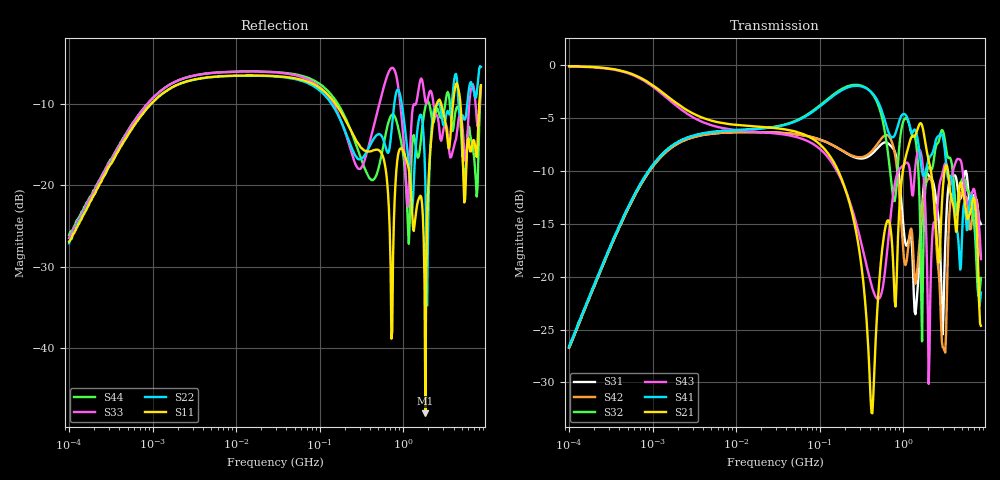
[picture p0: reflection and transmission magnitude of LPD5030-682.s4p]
# MHz S MA R 50
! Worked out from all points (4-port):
!   498 points, 100 kHz to 8.5 GHz, reference 50 ohm
!   strongest paths, dB at 100 kHz, 1.698 MHz, 29.49 MHz, 500.7 MHz, 8.5 GHz:
!     S21: -0.1, -3.3, -5.9, -21.9, -24.6
!     S41: -26.6, -7.6, -5.8, -3.5, -21.5
!     S43: -0.1, -3.5, -6.4, -22.1, -18.3
!     S32: -26.6, -7.6, -5.8, -3.7, -20.1
!     S42: -26.7, -7.8, -6.4, -7.4, -18.2
!     S31: -26.7, -7.8, -6.4, -7.8, -15.0
!   lowest |S11| = -48.1 dB at 1.84 GHz (marker M1), VSWR 1.01, Z = 50.2 - j0.32 ohm
!   |S11| at or under -10 dB: 156.2 MHz to 2.512 GHz (2.356 GHz wide, 177 % of centre); 2.857 GHz to 3.936 GHz (1.079 GHz wide, 31.8 % of centre); 4.843 GHz to 8.124 GHz (3.28 GHz wide, 50.6 % of centre)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
0.1  0.04505 82.2  0.9898 -2.7  0.04614 -95.9  0.0468 83.8
     0.9898 -2.7  0.04401 82.7  0.04667 84.2  0.04619 -96.0
     0.04614 -95.9  0.04667 84.2  0.04742 79.3  0.9877 -2.8
     0.0468 83.8  0.04619 -96.0  0.9877 -2.8  0.04945 82.5
110.9003  0.3844 -47.5  0.4068 -54.9  0.4393 115.5  0.6583 -2.5
          0.4068 -54.9  0.367 -45.4  0.6665 -4.1  0.4392 116.3
          0.4393 115.5  0.6665 -4.1  0.3834 -44.6  0.3878 -56.6
          0.6583 -2.5  0.4392 116.3  0.3878 -56.6  0.406 -45.4
417.0585  0.1627 -90.1  0.02271 137.5  0.3798 9.3  0.7447 -73.3
          0.02271 137.5  0.1845 -48.7  0.7412 -82.9  0.3911 9.6
          0.3798 9.3  0.7412 -82.9  0.2049 -19.7  0.09105 -145.0
          0.7447 -73.3  0.3911 9.6  0.09105 -145.0  0.1083 -63.6
1840.304  0.003934 -54.0  0.4283 110.0  0.3016 157.5  0.3115 107.0
          0.4283 110.0  0.1054 43.3  0.2661 143.7  0.2688 141.1
          0.3016 157.5  0.2661 143.7  0.3297 108.9  0.2085 71.3
          0.3115 107.0  0.2688 141.1  0.2085 71.3  0.3058 149.2
2476.442  0.3086 97.4  0.1662 16.4  0.2288 26.3  0.4462 27.9
          0.1662 16.4  0.3079 74.5  0.4162 42.8  0.1493 -5.8
          0.2288 26.3  0.4162 42.8  0.2714 25.6  0.1858 102.8
          0.4462 27.9  0.1493 -5.8  0.1858 102.8  0.2905 60.1
7080.634  0.1891 -131.7  0.2344 163.0  0.2438 157.9  0.215 149.1
          0.2344 163.0  0.3731 -169.8  0.1754 78.3  0.2351 167.0
          0.2438 157.9  0.1754 78.3  0.3873 -150.7  0.2589 164.4
          0.215 149.1  0.2351 167.0  0.2589 164.4  0.1464 -136.4
8500  0.416 -22.6  0.05865 2.2  0.1776 -35.5  0.08417 -7.7
      0.05865 2.2  0.5396 -40.9  0.09865 91.9  0.1237 -29.4
      0.1776 -35.5  0.09865 91.9  0.4051 -2.2  0.1211 -59.0
      0.08417 -7.7  0.1237 -29.4  0.1211 -59.0  0.4059 -7.9
